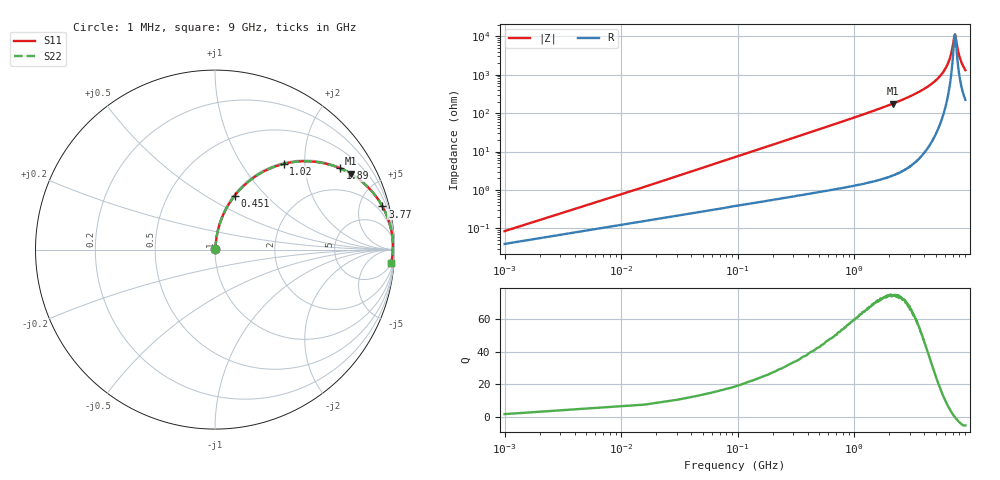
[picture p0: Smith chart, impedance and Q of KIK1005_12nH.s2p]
!version-3
!date-01.2023
!Series
# MHz S RI R 50
!Freq ReS11 ImS11 ReS21 ImS21 ReS12 ImS12 ReS22 ImS22
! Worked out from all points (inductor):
!   601 points, 1 MHz to 9 GHz, reference 50 ohm
!   read as one part in series: L = 12 nH near 46 MHz
!   highest Q = 74.3 at 2.15 GHz (marker M1), where L = 13.1 nH
!   self-resonance near 7.327 GHz
!   S11 on the Smith chart (normalised r, x): 1 MHz: 1.00, +0.00; 451 MHz: 1.02, +0.68; 1.02 GHz: 1.03, +1.57; 1.89 GHz: 1.04, +3.06; 3.77 GHz: 1.15, +7.72; 9 GHz: 5, -26
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1  0.000391 0.000753  0.9996 -0.000753  0.9996 -0.000753  0.000391 0.000753
61  0.00514 0.0456  0.9949 -0.0456  0.9949 -0.0456  0.00514 0.0456
106  0.0103 0.0788  0.9897 -0.0788  0.9897 -0.0788  0.0103 0.0788
166  0.0202 0.1221  0.9798 -0.1221  0.9798 -0.1221  0.0202 0.1221
241  0.0375 0.174  0.9625 -0.174  0.9625 -0.174  0.0375 0.174
451  0.1103 0.3012  0.8897 -0.3012  0.8897 -0.3012  0.1103 0.3012
691  0.2212 0.4052  0.7788 -0.4052  0.7788 -0.4052  0.2212 0.4052
1020  0.3833 0.4779  0.6167 -0.4779  0.6167 -0.4779  0.3833 0.4779
1520  0.5867 0.4853  0.4133 -0.4853  0.4133 -0.4853  0.5867 0.4853
1890  0.6976 0.4525  0.3024 -0.4525  0.3024 -0.4525  0.6976 0.4525
2150  0.7552 0.4233  0.2448 -0.4233  0.2448 -0.4233  0.7552 0.4233
3020  0.8787 0.319  0.1213 -0.319  0.1213 -0.319  0.8787 0.319
3770  0.933 0.2404  0.067 -0.2404  0.067 -0.2404  0.933 0.2404
4520  0.9632 0.1743  0.0368 -0.1743  0.0368 -0.1743  0.9632 0.1743
6020  0.9882 0.0704  0.0118 -0.0704  0.0118 -0.0704  0.9882 0.0704
6740  0.9912 0.0299  0.00877 -0.0299  0.00877 -0.0299  0.9912 0.0299
7290  0.9911 0.00171  0.00886 -0.00171  0.00886 -0.00171  0.9911 0.00171
7370  0.991 -0.00192  0.009 0.00192  0.009 0.00192  0.991 -0.00192
7520  0.9906 -0.00907  0.00937 0.00907  0.00937 0.00907  0.9906 -0.00907
7770  0.9898 -0.0209  0.0102 0.0209  0.0102 0.0209  0.9898 -0.0209
8070  0.9884 -0.0343  0.0116 0.0343  0.0116 0.0343  0.9884 -0.0343
9000  0.9821 -0.0725  0.0179 0.0725  0.0179 0.0725  0.9821 -0.0725
